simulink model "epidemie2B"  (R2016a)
settings: Solver=FixedStepDiscrete  StartTime=0.0  StopTime=1000  FixedStep=1  RelTol=1e-3
InitFcn:
  | init_epidemie
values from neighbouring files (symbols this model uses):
  alpha = 2e-6    (= 2e-06)    [init_epidemie.m]
  beta = 1    [init_epidemie.m]
  delta = 0.1    [init_epidemie.m]
  epsilon = 5e-3    (= 0.005)    [init_epidemie.m]
  gamma = 0.9    [init_epidemie.m]
  zeta = 4e-3    (= 0.004)    [init_epidemie.m]
undefined symbols (not defined in the file or in its folder): N0

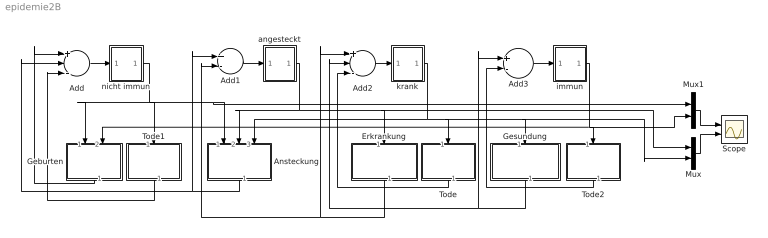
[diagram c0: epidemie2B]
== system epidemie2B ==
  Add : Sum  Inputs=+--
  Add1 : Sum  Inputs=+-
  Add2 : Sum  Inputs=+--
  Add3 : Sum  Inputs=+-
  Ansteckung : Subsystem
  Erkrankung : Subsystem
  Geburten : Subsystem
  Gesundung : Subsystem
  Mux : Mux  Inputs=2
  Mux1 : Mux  Inputs=2
  Scope : Scope  NumInputPorts=2
  Tode : Subsystem
  Tode1 : Subsystem
  Tode2 : Subsystem
  angesteckt : Subsystem
  immun : Subsystem
  krank : Subsystem
  nicht immun : Subsystem
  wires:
  Add/1 -> nicht immun/1(In)
  nicht immun/1(Out) -> Ansteckung/1(N), Mux1/1, Tode1/1(N), Geburten/1(N)
  immun/1(Out) -> Mux1/2, Tode2/1(I), Geburten/2(I)
  Geburten/1(b) -> Add/1
  angesteckt/1(Out) -> Ansteckung/2(A), Erkrankung/1(A), Mux/1
  krank/1(Out) -> Ansteckung/3(K), Tode/1(K), Gesundung/1(K), Mux/2
  Ansteckung/1(a) -> Add/2, Add1/1
  Add1/1 -> angesteckt/1(In)
  Erkrankung/1(k) -> Add2/1, Add1/2
  Add2/1 -> krank/1(In)
  Gesundung/1(g) -> Add3/1, Add2/2
  Tode/1(t) -> Add2/3
  Mux1/1 -> Scope/1
  Mux/1 -> Scope/2
  Add3/1 -> immun/1(In)
  Tode1/1(dn) -> Add/3
  Tode2/1(di) -> Add3/2

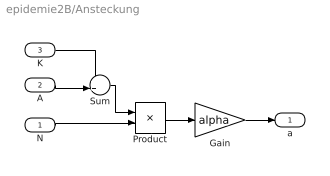
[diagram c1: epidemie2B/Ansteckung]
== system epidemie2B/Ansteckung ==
  N : Inport
  A : Inport  Port=2
  K : Inport  Port=3
  Gain : Gain  Gain=alpha
  Product : Product
  Sum : Sum  Inputs=++|
  a : Outport
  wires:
  Sum/1 -> Product/1
  Product/1 -> Gain/1
  K/1 -> Sum/1
  A/1 -> Sum/2
  Gain/1 -> a/1
  N/1 -> Product/2

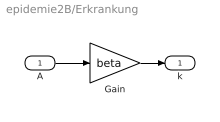
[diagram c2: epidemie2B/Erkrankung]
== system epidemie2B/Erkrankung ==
  A : Inport
  Gain : Gain  Gain=beta
  k : Outport
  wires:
  A/1 -> Gain/1
  Gain/1 -> k/1

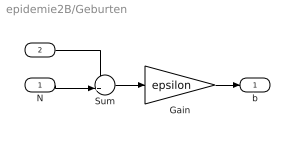
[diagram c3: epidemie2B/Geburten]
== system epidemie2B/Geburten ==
  N : Inport
  I : Inport  Port=2
  Gain : Gain  Gain=epsilon
  Sum : Sum  Inputs=++|
  b : Outport
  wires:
  Gain/1 -> b/1
  Sum/1 -> Gain/1
  N/1 -> Sum/2
  I/1 -> Sum/1

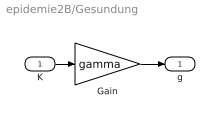
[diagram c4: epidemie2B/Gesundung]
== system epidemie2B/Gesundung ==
  K : Inport
  Gain : Gain  Gain=gamma
  g : Outport
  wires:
  Gain/1 -> g/1
  K/1 -> Gain/1

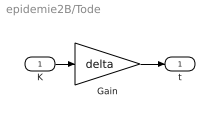
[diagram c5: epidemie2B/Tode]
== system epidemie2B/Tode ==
  K : Inport
  Gain : Gain  Gain=delta
  t : Outport
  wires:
  K/1 -> Gain/1
  Gain/1 -> t/1

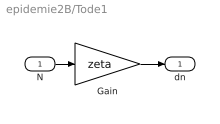
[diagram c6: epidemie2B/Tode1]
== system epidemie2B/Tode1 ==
  N : Inport
  Gain : Gain  Gain=zeta
  dn : Outport
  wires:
  Gain/1 -> dn/1
  N/1 -> Gain/1

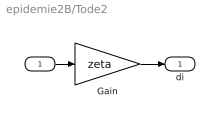
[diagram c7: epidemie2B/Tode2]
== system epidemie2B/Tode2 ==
  I : Inport
  Gain : Gain  Gain=zeta
  di : Outport
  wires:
  I/1 -> Gain/1
  Gain/1 -> di/1

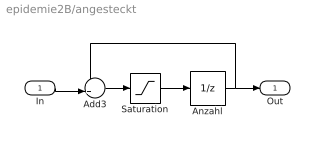
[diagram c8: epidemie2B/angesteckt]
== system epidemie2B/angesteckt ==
  In : Inport
  Add3 : Sum  Inputs=++|
  Anzahl : UnitDelay  InitialCondition=N0  SampleTime=-1
  Saturation : Saturate  UpperLimit=Inf  LowerLimit=0
  Out : Outport
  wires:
  Saturation/1 -> Anzahl/1
  Add3/1 -> Saturation/1
  Anzahl/1 -> Add3/1, Out/1
  In/1 -> Add3/2

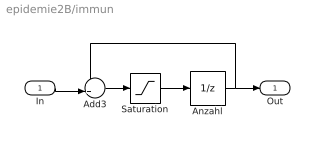
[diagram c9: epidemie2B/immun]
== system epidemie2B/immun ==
  In : Inport
  Add3 : Sum  Inputs=++|
  Anzahl : UnitDelay  InitialCondition=N0  SampleTime=-1
  Saturation : Saturate  UpperLimit=Inf  LowerLimit=0
  Out : Outport
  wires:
  In/1 -> Add3/2
  Anzahl/1 -> Out/1, Add3/1
  Add3/1 -> Saturation/1
  Saturation/1 -> Anzahl/1

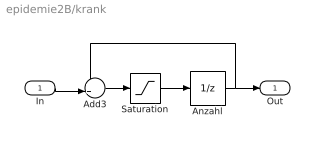
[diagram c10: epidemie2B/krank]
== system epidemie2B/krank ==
  In : Inport
  Add3 : Sum  Inputs=++|
  Anzahl : UnitDelay  InitialCondition=N0  SampleTime=-1
  Saturation : Saturate  UpperLimit=Inf  LowerLimit=0
  Out : Outport
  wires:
  Saturation/1 -> Anzahl/1
  Add3/1 -> Saturation/1
  Anzahl/1 -> Add3/1, Out/1
  In/1 -> Add3/2

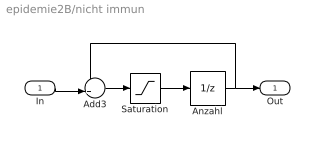
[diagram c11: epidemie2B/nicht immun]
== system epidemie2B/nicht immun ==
  In : Inport
  Add3 : Sum  Inputs=++|
  Anzahl : UnitDelay  InitialCondition=N0  SampleTime=-1
  Saturation : Saturate  UpperLimit=Inf  LowerLimit=0
  Out : Outport
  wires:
  In/1 -> Add3/2
  Anzahl/1 -> Out/1, Add3/1
  Add3/1 -> Saturation/1
  Saturation/1 -> Anzahl/1
